(* 	
	Program Name: 	ACS_CMD_HOME_HERE
	Purpose:		Copy Home Here Command to ACS Drive Output Command Register
	When Executed:	Declares current position home
*)
PROGRAM ACS_CMD_HOME_HERE
VAR_IN_OUT
	Axis:ACS_DRIVE_TYPE;
END_VAR
VAR
	_command:	USINT	:= ACS_COMMANDS.HOME_HERE;
END_VAR

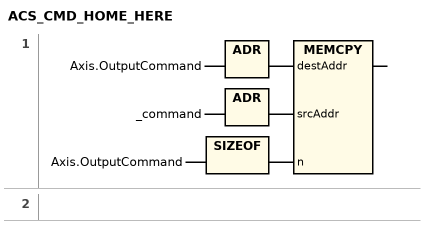
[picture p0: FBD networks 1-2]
// NETWORK 1
MEMCPY(destAddr := ADR(Axis.OutputCommand), srcAddr := ADR(_command), n := SIZEOF(Axis.OutputCommand));

// NETWORK 2

END_PROGRAM
